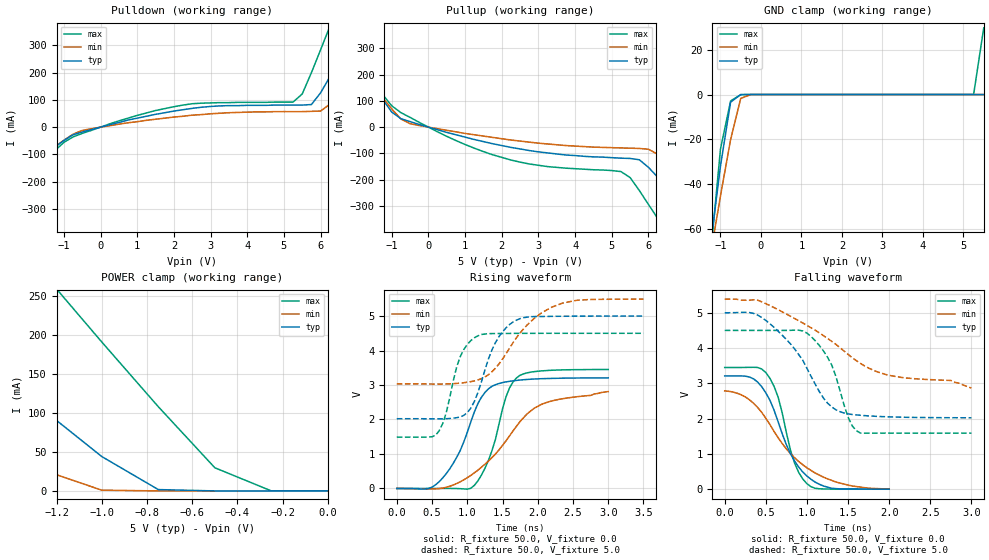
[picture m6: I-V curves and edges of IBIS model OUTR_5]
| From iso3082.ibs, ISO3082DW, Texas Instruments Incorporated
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[Model]   OUTR_5
Model_type   3-state
| Signals   R
Vmeas = 2.2V   |Reference voltage for timing measurements
Cref = 15pF   |Timing specification test load capacitance value
Vref = 0   |Timing specification test load voltage; GND
| variable   typ   min   max
C_comp   2.1pF   1.7pF   2.5pF
|   typ   min   max
[Temperature Range]   25.0   -40   85
[Voltage range]   5.0V   5.5V   4.5V
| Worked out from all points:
|   slope of the pulldown table from 0 to 0.75 V, typ, clamps not added: 28.8 ohm
|   slope of the pullup table from 0 to 0.75 V, typ, clamps not added: 25.9 ohm
|   GND clamp passes 1 mA (typ) near -0.57 V on its own axis
|   POWER clamp passes 1 mA (typ) near -0.64 V on its own axis
|   rising waveform, R_fixture 50.0, V_fixture 0.0: 20-80 % time 405ps typ, 730ps min, 296ps max; typ from 0.001 V to 3.21 V
|   falling waveform, R_fixture 50.0, V_fixture 0.0: 20-80 % time 356ps typ, 598ps min, 234ps max; typ from 3.21 V to 0.001 V
|   rising waveform, R_fixture 50.0, V_fixture 5.0: 20-80 % time 332ps typ, 579ps min, 234ps max; typ from 2.02 V to 5 V
|   falling waveform, R_fixture 50.0, V_fixture 5.0: 20-80 % time 509ps typ, 996ps min, 281ps max; typ from 5 V to 2.02 V
[Pulldown]
|   Voltage   I(typ)  I(min)  I(max)
-5.5V     -720mA     -549mA     -979mA
-4V       -488mA     -379mA     -657mA
-2.75V    -296mA     -239mA     -390mA
-1.25V    -74mA      -73mA      -87mA
-500mV    -18mA      -12mA      -23mA
2.25V     64mA       40mA       81mA
5.25V     81mA       57mA       92mA
5.75V     83mA       58mA       200mA
6.25V     184mA      84mA       369mA
7V        370mA      213mA      628mA
8V        624mA      398mA      979mA
11V       1.431A     985mA      2.089A
[Pullup]
|   Voltage   I(typ)  I(min)  I(max)
| Note that the[Pullup]voltage table is referenced to Vcc
| and is calculated using Vtable=Vcc - Vmeasured.
-5.5V     1.17A      899mA      1.572A
-2.75V    475mA      386mA      620mA
-2.25V    350mA      293mA      448mA
-2V       288mA      247mA      363mA
-1.25V    106mA      112mA      124mA
-750mV    32mA       31mA       55mA
2.25V     -77mA      -49mA      -125mA
5.25V     -118mA     -79mA      -169mA
6.5V      -229mA     -129mA     -401mA
7.5V      -385mA     -241mA     -618mA
8.75V     -581mA     -384mA     -891mA
11V       -936mA     -644mA     -1.385A
[GND_clamp]
|   Voltage   I(typ)   I(min)   I(max)
| Outputs in High Impedance (off)
-5.5V     -720mA     -549mA     -979mA
-1.25V    -67.7mA    -71.9mA    -72.6mA
-1V       -31.9mA    -45.2mA    -24.3mA
-750mV    -3.4mA     -20.1mA    -2.87mA
-500mV    -16.7uA    -1.73mA    -51.5uA
-250mV    -5.22nA    -2.79uA    -3.69nA
5.25V     104pA      2.34nA     13.2uA
5.5V      149nA      3.67nA     29.7mA
[POWER_clamp]
|   Voltage  I(typ)   I(min)   I(max)
| Note that the [POWER_clamp] voltage table is referenced to Vcc
| and is calculated using Vtable = Vcc - Vmeasured.
| Outputs in Tri-state.
-5.5V     1.17A      806mA      1.74A
-2.75V    475mA      293mA      791mA
-2.5V     412mA      246mA      705mA
-2V       287mA      155mA      533mA
-1.75V    225mA      110mA      447mA
-1.5V     163mA      66.4mA     361mA
-1.25V    102mA      25.7mA     276mA
-1V       44.1mA     970uA      191mA
-750mV    1.74mA     1.18uA     108mA
-500mV    149nA      3.67nA     29.7mA
-250mV    104pA      2.34nA     13.2uA
0V        83.4pA     2.25nA     534pA
[Ramp]
|   typ   min   max
dV/dt_r   1.88V/.33ns   1.48V/.58ns   1.81V/.23ns
dV/dt_f   1.92V/.36ns   1.67V/.60ns   2.07V/.23ns
R_load = 50
[Rising Waveform]
R_fixture = 50.0
V_fixture = 0.0
C_fixture = 0p
L_fixture = 0n
|   V(typ)   V(min)   V(max)
0s        581.6uV    -629.5uV   5.172nV
450ps     -1.459mV   -14.21mV   -4.334uV
650ps     300.8mV    10.64mV    182.2uV
900ps     1.098V     192.7mV    -7.155mV
1.05ns    1.929V     378.3mV    4.684mV
1.35ns    2.962V     896.3mV    1.094V
1.55ns    3.091V     1.382V     2.66V
1.75ns    3.145V     1.944V     3.283V
2.1ns     3.186V     2.475V     3.416V
3ns       3.207V     2.81V      3.45V
[Falling Waveform]
R_fixture = 50.0
V_fixture = 0.0
C_fixture = 0p
L_fixture = 0n
|   V(typ)   V(min)   V(max)
0s        3.209V     2.786V     3.45V
300ps     3.18V      2.535V     3.453V
400ps     3.038V     2.318V     3.45V
500ps     2.731V     2.009V     3.307V
650ps     1.908V     1.458V     2.607V
800ps     1.003V     1.007V     1.102V
850ps     797.5mV    890mV      739.7mV
1ns       372mV      605.1mV    154.7mV
1.3ns     25.67mV    249.5mV    3.199mV
2ns       1.251mV    5.348mV    18.15uV
[Rising Waveform]
R_fixture = 50.0
V_fixture = 5.0
V_fixture_min = 5.5
V_fixture_max = 4.5
C_fixture = 0p
L_fixture = 0n
|   V(typ)   V(min)  V(max)
0s        2.022V     3.032V     1.489V
600ps     2.019V     3.028V     1.666V
700ps     2.022V     3.03V      2.186V
900ps     2.073V     3.054V     3.823V
1.15ns    2.777V     3.147V     4.426V
1.4ns     4.231V     3.488V     4.493V
1.7ns     4.884V     4.38V      4.498V
2.05ns    4.988V     5.087V     4.5V
2.35ns    4.994V     5.375V     4.5V
3.5ns     5V         5.493V     4.5V
[Falling Waveform]
R_fixture = 50.0
V_fixture = 5.0
V_fixture_min = 5.25
V_fixture_max = 4.75
C_fixture = 0p
L_fixture = 0n
|   V(typ)   V(min)  V(max)
0s        5V         5.389V     4.5V
450ps     4.867V     5.311V     4.5V
800ps     4.118V     4.902V     4.503V
1ns       3.426V     4.642V     4.424V
1.25ns    2.441V     4.273V     3.742V
1.4ns     2.199V     4.014V     2.81V
1.5ns     2.135V     3.822V     2.041V
1.65ns    2.095V     3.565V     1.59V
2ns       2.05V      3.225V     1.589V
3ns       2.023V     2.866V     1.589V
